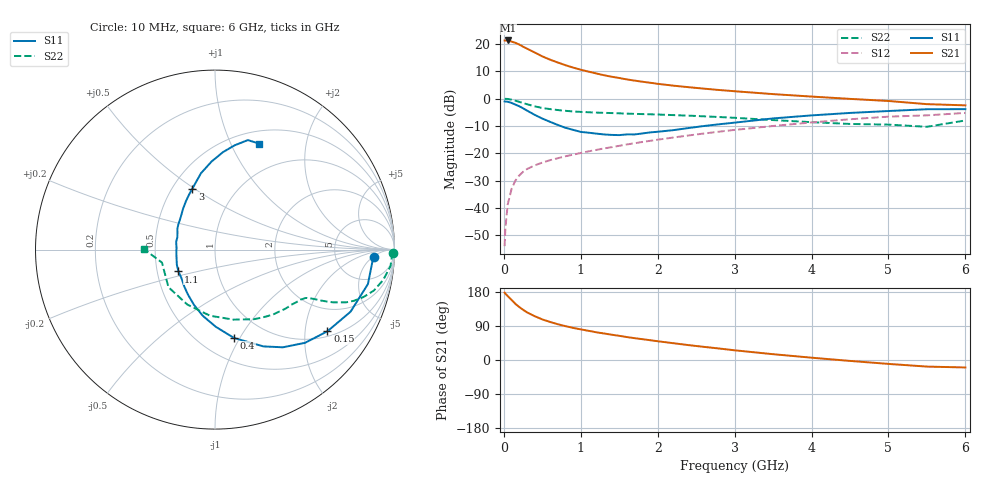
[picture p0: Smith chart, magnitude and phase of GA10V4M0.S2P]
! Infineon Technologies  Discrete & RF Semiconductors
! BF775
! Si NPN RF Bipolar Junction Transistor in SOT23
! VCE = 10 V  IC = 4 mA
! Common Emitter S-Parameters:  May  1996
# GHz  S  MA  R  50
!  f  S11  S21  S12  S22
! GHz  MAG  ANG  MAG  ANG  MAG  ANG  MAG  ANG
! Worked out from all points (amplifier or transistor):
!   36 points, 10 MHz to 6 GHz, reference 50 ohm
!   highest |S21| = 21.2 dB at 50 MHz (marker M1)
!   |S21| within 3 dB of that: start of sweep to 301 MHz
!   unconditionally stable (mu >= 1): 936.1 MHz to 3.005 GHz
!   at 250 MHz: K = 0.41, MSG = 22.9 dB, |S12| = -26.8 dB
!   at 1.4 GHz: K = 1.10, MAG = 10.9 dB, |S12| = -17.8 dB
!   at 6 GHz: K = 0.89, MSG = 1.4 dB, |S12| = -5.3 dB
!   S11 on the Smith chart (normalised r, x): 10 MHz: 14, -5; 150 MHz: 1.15, -2.63; 400 MHz: 0.72, -0.95; 1.1 GHz: 0.64, -0.17; 3 GHz: 0.63, +0.49; 6 GHz: 0.64, +1.29
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0.01  0.884 -2.6  11.49 177.6  0.002 88.5  0.9946 -1.0
0.02  0.8783 -5.0  11.46 175.1  0.0042 89.1  0.9865 -2.1
0.05  0.8734 -12.7  11.51 168.9  0.0115 84.4  0.9821 -5.4
0.1  0.8308 -24.6  10.98 158.8  0.0221 75.8  0.9519 -10.3
0.15  0.7744 -36.0  10.42 148.1  0.0316 71.1  0.9136 -14.5
0.2  0.722 -46.0  9.707 139.9  0.0392 66.8  0.8687 -17.7
0.25  0.6629 -55.2  8.855 132.5  0.0457 63.3  0.8255 -20.2
0.3  0.6032 -63.4  8.164 125.9  0.0513 61.1  0.7876 -21.9
0.4  0.5039 -77.8  6.953 115.7  0.0598 58.0  0.7195 -24.1
0.5  0.4302 -89.4  5.887 107.1  0.0674 56.4  0.6706 -25.3
0.6  0.3753 -100.4  5.137 100.5  0.0746 56.0  0.6407 -26.0
0.7  0.3292 -110.9  4.56 94.5  0.081 56.1  0.6159 -26.5
0.9  0.2675 -129.8  3.68 84.7  0.0942 56.8  0.5798 -27.7
1.1  0.2373 -149.1  3.102 77.1  0.1081 57.2  0.5608 -29.4
1.3  0.2207 -165.8  2.669 70.0  0.1222 57.6  0.5472 -31.3
1.6  0.2208 168.7  2.232 60.5  0.1447 57.9  0.5299 -34.8
2.2  0.2638 136.2  1.721 44.4  0.1934 56.4  0.4978 -43.9
3  0.3623 110.4  1.358 25.6  0.2667 51.2  0.4442 -60.8
3.5  0.4326 100.4  1.204 15.3  0.3146 46.4  0.4036 -75.2
4.5  0.5449 85.3  0.985 -2.4  0.4176 34.9  0.3428 -116.7
5.5  0.637 73.3  0.789 -17.4  0.4923 19.3  0.3042 -166.3
6  0.6395 67.5  0.75 -19.7  0.5457 15.0  0.397 179.5
